FUNCTION_BLOCK FB_WithProperties
VAR
    _value : INT;
    _name : STRING(80);
    _enabled : BOOL;
END_VAR

PROPERTY PUBLIC Value : INT
GET
VAR
    temp : INT;
END_VAR
temp := _value;
Value := temp;
END_GET
SET
_value := Value;
END_SET
END_PROPERTY

PROPERTY Name : STRING(80)
GET
Name := _name;
END_GET
SET
_name := Name;
END_SET
END_PROPERTY

PROPERTY Enabled : BOOL
GET
Enabled := _enabled;
END_GET
END_PROPERTY

METHOD DoWork : BOOL
IF _enabled THEN
    _value := _value + 1;
    DoWork := TRUE;
END_IF
END_METHOD

END_FUNCTION_BLOCK
